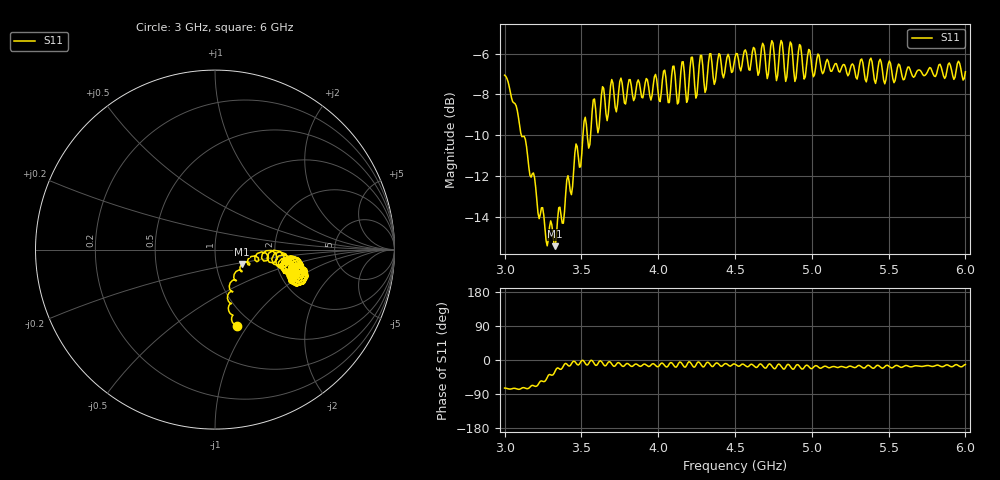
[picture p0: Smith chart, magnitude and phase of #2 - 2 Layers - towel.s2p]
!  02/07/2025  16:39:35
! Ref Plane: 0.000 mm
# MHZ S MA R  50
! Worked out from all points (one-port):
!   401 points, 3 GHz to 6 GHz, reference 50 ohm
!   lowest |S11| = -15.5 dB at 3.33 GHz (marker M1), VSWR 1.41, Z = 66.4 - j11 ohm
!   |S11| at or under -10 dB: 3.109 GHz to 3.51 GHz (401 MHz wide, 12.1 % of centre); 3.538 GHz to 3.56 GHz (21.5 MHz wide, 0.606 % of centre)
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3000  0.4436 -74.1
3270  0.1742 -52.2
3330  0.1688 -28.6
3375  0.1923 -21.4
3525  0.3497 -8.8
3750  0.4281 -9.0
4095  0.4661 -10.5
4125  0.3769 -14.7
4155  0.4779 -9.8
4185  0.3803 -14.2
4215  0.4904 -9.6
4245  0.3896 -14.2
4275  0.4958 -9.7
4305  0.4023 -13.7
4335  0.5003 -9.9
4500  0.49 -10.9
4695  0.4962 -21.4
4725  0.485 -10.1
4755  0.4993 -23.1
4785  0.482 -10.6
4815  0.4991 -23.9
4845  0.4767 -11.3
4875  0.4962 -24.2
4905  0.4704 -12.1
4935  0.4944 -23.8
5250  0.4597 -16.1
5625  0.4641 -15.7
6000  0.4521 -11.8
